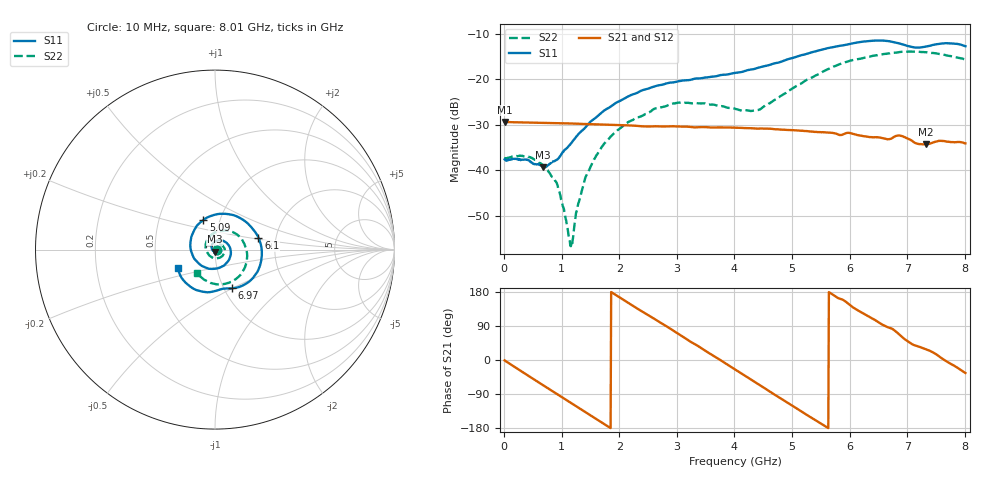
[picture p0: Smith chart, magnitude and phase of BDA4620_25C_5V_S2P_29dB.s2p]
!Agilent Technologies,E5071B,MY42404982,A.09.10
!Date: Wed May 06 09:04:46 2026
!Data & Calibration Information:
!Freq	S11:SOLT2(ON)	S21:SOLT2(ON)	S12:SOLT2(ON)	S22:SOLT2(ON)
# Hz S RI R 50
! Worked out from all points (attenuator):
!   801 points, 10 MHz to 8.01 GHz, reference 50 ohm
!   highest |S21| = -29.38 dB at 10 MHz (marker M1); lowest = -34.3 dB at 7.32 GHz (marker M2)
!   lowest |S11| = -39.4 dB at 680 MHz (marker M3), VSWR 1.02, Z = 49.9 - j1.06 ohm
!   |S11| at or under -10 dB: start of sweep to end of sweep
!   |S22| runs from -56.7 to -13.9 dB; largest |S21 - S12| = 0.00017
!   S11 on the Smith chart (normalised r, x): 10 MHz: 1.03, -0.00; 5.09 GHz: 0.83, +0.28; 6.1 GHz: 1.62, +0.23; 6.97 GHz: 1.09, -0.50; 8.01 GHz: 0.65, -0.14
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1e7  0.0131 -0.000825  0.034 -0.000678  0.034 -0.00071  0.0135 -0.000455
4.1e8  0.00845 -0.0098  0.0255 -0.0217  0.0255 -0.0218  0.0134 -0.00454
6.8e8  -0.00132 -0.0106  0.0131 -0.0305  0.0131 -0.0306  0.0092 -0.00649
9.3e8  -0.0122 -0.00503  -0.000632 -0.0329  -0.000681 -0.033  0.0036 -0.00576
1.16e9  -0.0183 0.00694  -0.0129 -0.0299  -0.013 -0.0299  -0.00127 -0.000724
1.19e9  -0.0188 0.00885  -0.0144 -0.0292  -0.0145 -0.0292  -0.00167 0.000107
1.35e9  -0.0187 0.0196  -0.0215 -0.0241  -0.0216 -0.0241  -0.00323 0.00495
1.53e9  -0.0135 0.0325  -0.0275 -0.0165  -0.0275 -0.0165  -0.00295 0.0114
1.77e9  0.00172 0.0465  -0.0314 -0.00443  -0.0314 -0.0044  0.00115 0.0204
2.14e9  0.0387 0.0507  -0.0276 0.0144  -0.0277 0.0144  0.0168 0.0287
2.68e9  0.0854 0.00581  -0.00632 0.0297  -0.00628 0.0297  0.0443 0.0191
3.08e9  0.0794 -0.0543  0.0133 0.0271  0.0134 0.0271  0.0549 -0.00754
4.01e9  -0.0776 -0.088  0.0266 -0.0124  0.0266 -0.0124  -0.0106 -0.0463
4.42e9  -0.134 -0.00552  0.0126 -0.0258  0.0125 -0.0258  -0.0444 -0.0126
5.09e9  -0.065 0.1654  -0.0171 -0.0213  -0.0172 -0.0214  -0.0198 0.0832
5.35e9  0.0148 0.1978  -0.0238 -0.0119  -0.0238 -0.0118  0.0232 0.102
6.1e9  0.2421 0.0662  -0.0174 0.0175  -0.0175 0.0175  0.1593 0.0414
6.68e9  0.1974 -0.1724  0.00162 0.0219  0.00161 0.0219  0.1697 -0.0894
6.97e9  0.0962 -0.2155  0.0136 0.0184  0.0136 0.0183  0.1305 -0.1524
7.32e9  0.0127 -0.2277  0.0169 0.00919  0.0169 0.0092  0.0491 -0.1921
7.66e9  -0.1116 -0.2223  0.0208 -0.000558  0.0208 -0.000566  -0.0346 -0.1811
8.01e9  -0.2055 -0.1044  0.0163 -0.0111  0.0163 -0.011  -0.1027 -0.1284
